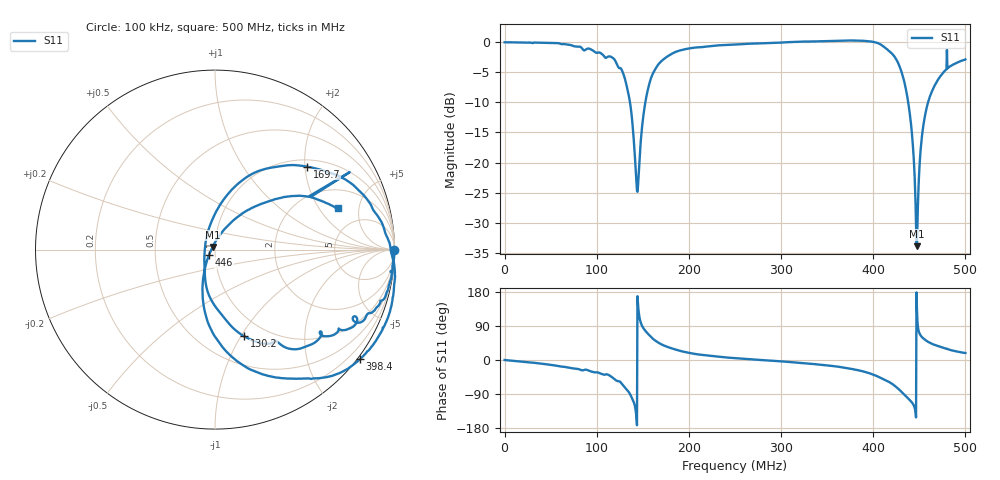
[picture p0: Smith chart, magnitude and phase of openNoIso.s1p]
# Hz S RI R 50.0
! written by SimSmith version 18.3h
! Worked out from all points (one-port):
!   1000 points, 100 kHz to 500 MHz, reference 50 ohm
!   lowest |S11| = -33.9 dB at 447.5 MHz (marker M1), VSWR 1.04, Z = 48.7 + j1.47 ohm
!   |S11| at or under -10 dB: 136.1 MHz to 152.8 MHz (16.64 MHz wide, 11.5 % of centre); 438 MHz to 459.5 MHz (21.5 MHz wide, 4.79 % of centre)
!   S11 on the Smith chart (normalised r, x): 100 kHz: open; 130.2 MHz: 0.79, -1.03; 169.7 MHz: 1.16, +2.06; 398.4 MHz: -0.06, -2.98; 446 MHz: 0.93, -0.06; 500 MHz: 3.14, +3.00
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100000  0.9998 -0.000417
6.265005e7  0.9214 -0.2857
1.131905e8  0.5861 -0.4886
1.252001e8  0.3317 -0.5105
1.302041e8  0.163 -0.4832
1.367093e8  -0.0127 -0.2949
1.422137e8  -0.0594 -0.0663
1.442153e8  -0.0559 0.0114
1.502201e8  0.0171 0.2307
1.547237e8  0.1204 0.3599
1.697357e8  0.5147 0.4619
1.877502e8  0.7589 0.3685
2.503002e8  0.9533 0.0822
3.128503e8  1.001 -0.1044
3.754003e8  0.9536 -0.4036
3.984187e8  0.8078 -0.6096
4.229383e8  0.2951 -0.7034
4.314451e8  0.041 -0.5422
4.379504e8  -0.0635 -0.3105
4.42454e8  -0.0637 -0.1455
4.459568e8  -0.0339 -0.03
4.47458e8  -0.0133 0.0151
4.489592e8  0.00938 0.0563
4.514612e8  0.055 0.1161
4.534628e8  0.0936 0.1547
4.609688e8  0.2398 0.2475
4.77482e8  0.4938 0.298
5e8  0.6833 0.2292
